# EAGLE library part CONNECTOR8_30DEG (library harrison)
8-pin connector turned 30 degrees
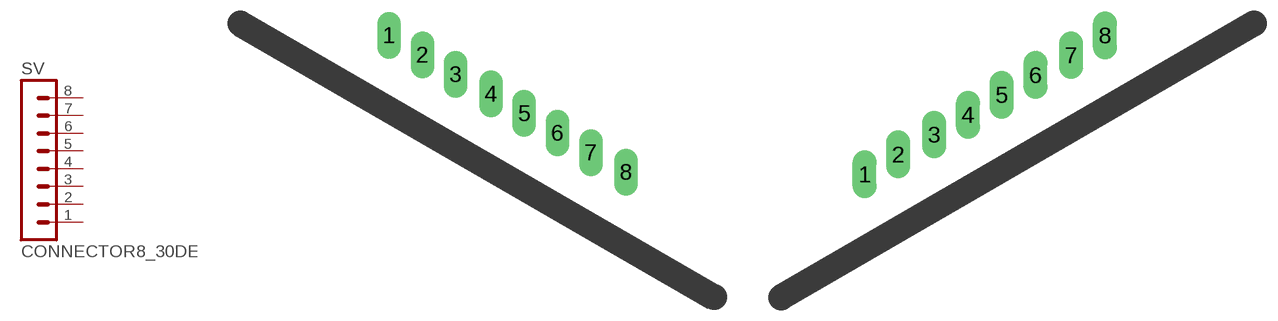
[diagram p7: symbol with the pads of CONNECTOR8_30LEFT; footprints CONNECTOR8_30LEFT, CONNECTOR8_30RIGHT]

Designator prefix SV

## CONNECTOR8_30DEGLEFT  [CONNECTOR8_30LEFT]
1  1  pas
2  2  pas
3  3  pas
4  4  pas
5  5  pas
6  6  pas
7  7  pas
8  8  pas

## CONNECTOR8_30DEGRIGHT  [CONNECTOR8_30RIGHT]
Pads as for CONNECTOR8_30LEFT

## Footprint CONNECTOR8_30LEFT (pad centres in mm)
drill 1.016 long: 1 -15.367,8.89; 2 -13.208,7.62; 3 -11.049,6.35; 4 -8.763,5.08; 5 -6.604,3.81; 6 -4.445,2.54; 7 -2.286,1.27; 8 0,0

## Footprint CONNECTOR8_30RIGHT (pad centres in mm)
drill 1.016 long: 1 0,0; 2 2.159,1.27; 3 4.445,2.54; 4 6.604,3.81; 5 8.763,5.08; 6 10.922,6.35; 7 13.208,7.62; 8 15.367,8.89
